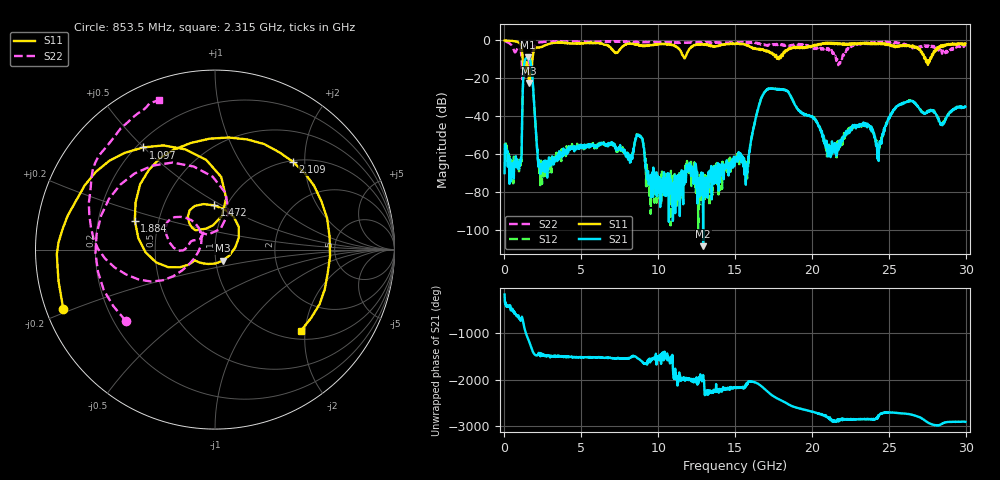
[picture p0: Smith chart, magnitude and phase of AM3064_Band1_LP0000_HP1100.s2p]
# Hz S DB R 50.0
!freq dBS11 angS11 dBS21 angS21 dBS12 angS12 dBS22 angS22
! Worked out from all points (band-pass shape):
!   1600 points, 10 MHz to 29.98 GHz, reference 50 ohm
!   highest |S21| = -9.00 dB at 1.528 GHz (marker M1); lowest = -108.6 dB at 12.92 GHz (marker M2)
!   |S21| within 3 dB of the highest: 1.296 GHz to 1.715 GHz (418.6 MHz wide, 27.8 % of centre)
!   lowest |S11| = -22.4 dB at 1.603 GHz (marker M3), VSWR 1.16, Z = 54 - j6.77 ohm
!   |S11| at or under -10 dB: 1.187 GHz to 1.822 GHz (635.6 MHz wide, 42.3 % of centre); 27.4 GHz to 27.68 GHz (284 MHz wide, 1.03 % of centre)
!   |S22| runs from -21.8 to -0.2 dB; largest |S21 - S12| = 0.0051
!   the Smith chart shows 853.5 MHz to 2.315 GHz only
!   S11 on the Smith chart (normalised r, x): 853.5 MHz: 0.05, -0.19; 1.097 GHz: 0.23, +0.50; 1.472 GHz: 0.88, +0.46; 1.884 GHz: 0.37, +0.15; 2.109 GHz: 1.02, +1.75; 2.315 GHz: 1.19, -1.90
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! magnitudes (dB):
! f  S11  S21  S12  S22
! 10 MHz  0.0  -70.0  -54.4  -0.2
! 853.5 MHz  -0.8  -65.0  -65.0  -3.9
! 1.097 GHz  -3.1  -62.7  -64.0  -7.8
! 1.472 GHz  -12.2  -9.1  -9.0  -10.4
! 1.528 GHz  -14.7  -9.0  -9.0  -10.8
! 1.603 GHz  -22.4  -9.4  -9.3  -14.7
! 1.884 GHz  -6.5  -27.6  -27.5  -4.2
! 2.109 GHz  -3.7  -56.3  -54.9  -1.6
! 2.315 GHz  -3.6  -67.3  -66.9  -1.0
! 5.015 GHz  -1.4  -55.4  -56.4  -0.7
! 8.745 GHz  -2.6  -50.2  -49.9  -1.1
! 10 GHz  -2.0  -77.3  -73.5  -0.9
! 12.92 GHz  -2.2  -108.6  -76.3  -1.1
! 15 GHz  -1.8  -63.5  -63.8  -1.3
! 15.77 GHz  -2.6  -69.2  -68.5  -1.0
! 17.14 GHz  -5.8  -25.5  -25.6  -2.7
! 19.99 GHz  -3.4  -40.2  -40.4  -3.4
! 21.1 GHz  -1.7  -57.7  -54.4  -5.3
! 23.36 GHz  -1.6  -45.1  -44.2  -1.9
! 24.36 GHz  -1.7  -57.5  -56.5  -1.5
! 25 GHz  -2.1  -40.7  -41.6  -1.1
! 29.98 GHz  -1.7  -35.0  -35.4  -3.2
